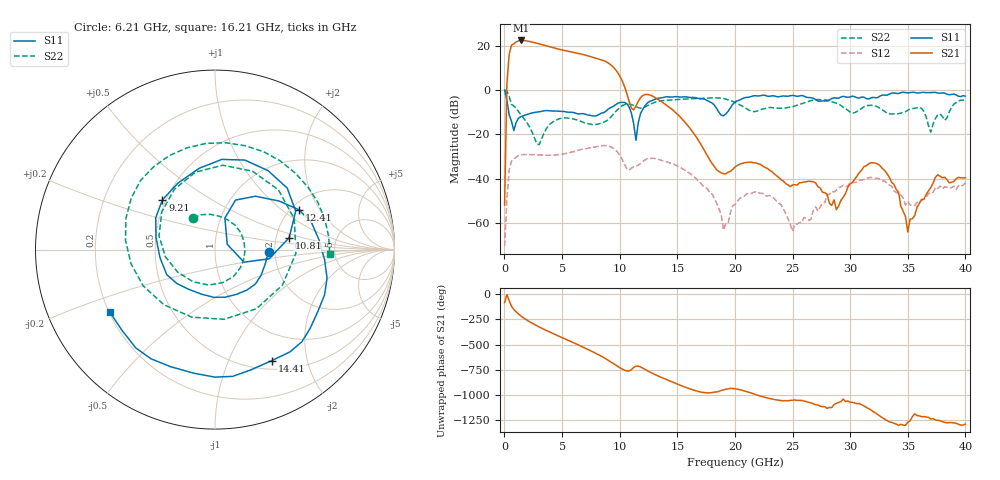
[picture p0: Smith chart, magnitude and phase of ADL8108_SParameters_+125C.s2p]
! Analog Devices, Inc.
! Device:	ADL8108 SN8565
! Description:	"GaAs, pHEMT, MMIC, Low Noise Amplifier, 1.5 GHz to 6 GHz"
! Conditions:	Vdd = 5.0 V
!		Idq = 90 mA
!  Rbias = 1270 Ohm
!		Pin = -25 dBm
!		Operating Temperature = +125 C (at package bottom)
! Board loss de-embedded from S21 magnitude.  All other RF measurements reference to RF coaxial connector.
! Frequency (GHz)	S11_Mag (dB)	S11_Phase (deg)	S21_Mag (dB)	S21_Phase (deg)	S12_Mag (dB)	S12_Phase (deg)	S22_Mag (dB)	S22_Phase (deg)
#  GHZ  S  DB  R 50
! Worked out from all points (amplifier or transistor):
!   201 points, 10 MHz to 40 GHz, reference 50 ohm
!   highest |S21| = 22.4 dB at 1.41 GHz (marker M1)
!   |S21| within 3 dB of that: 566.7 MHz to 4.04 GHz (3.473 GHz wide, 151 % of centre)
!   unconditionally stable (mu >= 1): 14.45 MHz to end of sweep
!   at 6.61 GHz: K = 1.57, MAG = 17.1 dB, |S12| = -26.8 dB
!   at 20 GHz: K = 5261.67, MAG = -31.8 dB, |S12| = -51.6 dB
!   at 40 GHz: K = 1709.26, MAG = -34.2 dB, |S12| = -41.7 dB
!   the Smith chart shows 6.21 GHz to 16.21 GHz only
!   S11 on the Smith chart (normalised r, x): 6.21 GHz: 1.85, -0.05; 9.21 GHz: 0.48, +0.32; 10.81 GHz: 2.37, +0.38; 12.41 GHz: 2.19, +1.33; 14.41 GHz: 0.61, -1.46; 16.21 GHz: 0.20, -0.26
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0.01  -0.03 -5.2  -51.82 -85.2  -70.35 -140.2  0.01 -2.4
0.21  -4.64 -95.0  3.03 -5.4  -49.13 -174.0  -0.46 -49.1
0.41  -11.24 -128.7  16.25 -67.3  -35.92 127.3  -3.01 -96.0
0.61  -14.03 -146.1  20.25 -121.4  -32.03 79.1  -6.43 -118.6
1.01  -14.58 -131.0  21.69 -176.0  -30.21 35.2  -8.20 -163.0
1.41  -11.98 -156.3  22.39 144.2  -29.20 6.8  -10.96 156.8
2.21  -10.52 166.4  21.89 83.5  -29.09 -32.6  -16.92 89.5
3.41  -9.33 121.9  20.28 11.6  -29.35 -72.6  -19.60 -86.0
4.81  -9.52 67.2  18.34 -61.4  -29.00 -110.3  -12.81 -164.7
6.21  -10.47 -2.1  16.78 -132.5  -27.44 -151.3  -13.30 124.6
6.81  -10.59 -40.3  16.07 -164.7  -26.64 -172.3  -14.52 83.2
8.21  -10.93 -138.4  13.96 117.0  -25.21 130.6  -15.20 -36.6
9.21  -7.88 136.6  11.45 50.3  -25.55 76.3  -12.29 -148.8
10.81  -7.57 9.1  -5.00 -40.6  -36.04 33.9  -6.28 43.3
12.41  -5.73 25.5  -1.95 -38.5  -30.90 4.9  -6.97 -153.1
13.41  -3.60 -22.5  -4.42 -94.3  -31.28 -42.1  -4.95 137.2
14.41  -3.16 -62.8  -8.11 -142.2  -32.96 -84.1  -4.46 84.4
16.21  -3.33 -149.3  -17.98 138.2  -37.96 -159.7  -3.88 -2.4
20.2  -4.84 149.4  -33.93 139.9  -50.49 -167.3  -6.05 -177.8
26.8  -3.67 -83.0  -41.27 -3.9  -54.16 119.5  -4.54 109.2
33.4  -1.83 107.5  -39.23 176.4  -42.72 -127.5  -10.65 108.1
40  -2.70 -12.5  -39.52 154.5  -41.72 132.8  -4.45 -37.9
